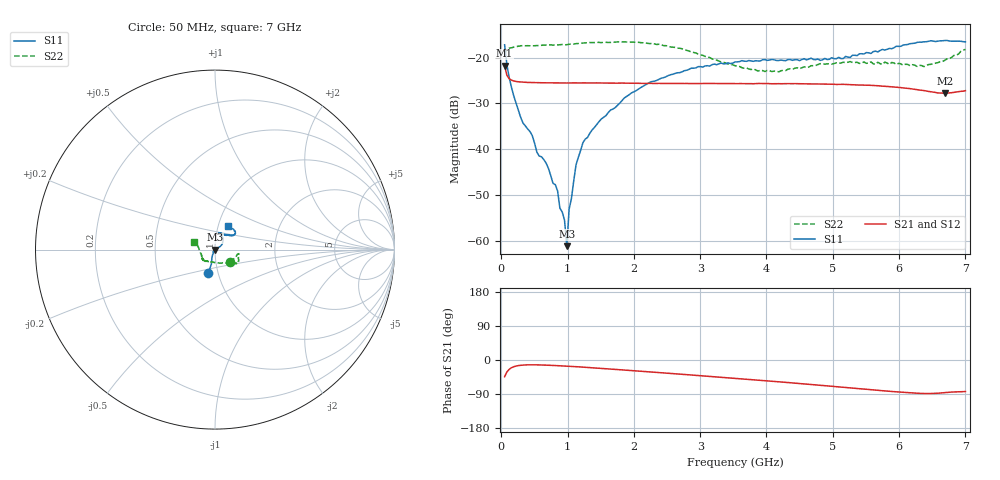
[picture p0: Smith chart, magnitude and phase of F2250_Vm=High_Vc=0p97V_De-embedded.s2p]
! Integrated Device Technology
! Corporate Headquarters
! 6024 Silver Creek Valley Road
! San Jose, CA 95138  USA
! Phone:  1-408-284-8200
! Toll Free:  1-800-223-1366
! Webpage:  http://www.idt.com/
! Timing and RF Division
! 515 Groton Road, Suite 102
! Westford, MA 01886-6024
! Device:  F2250
! Description: Voltage Variable RF Attenuator
! Frequency:  50.0 -  6000.00 MHz
! Package:  3x3 mm Thin QFN Plastic Package: 16 pin
! Ports:  2 RF, 3 DC
!  Pin  1  = GND
!  Pin  2  = NC
!  Pin  3  = RF1  = Port 1
!  Pin  4  = NC
!  Pin  5  = GND
!  Pin  6  = GND
!  Pin  7  = GND
!  Pin  8  = GND
!  Pin  9  = NC
!  Pin 10  = RF2  = Port 2
!  Pin 11  = NC
!  Pin 12  = GND
!  Pin 13  = GND
!  Pin 14  = VCNTRL
!  Pin 15  = VDD
!  Pin 16  = VMODE
! Vcntrl:  0.970 Volts
! Vmode:  +3.300 Volts
! Vdd:  +3.30  Volts
! Current:  1.324 mA
! Data:  The device was measured on a the F2250 evaluation board which has
!  individual transmission lines to the RF pins.  Data was collected
!  using a calibrated network analyzer.  The evaluation board was
!  de-embedded using a TRL calibration technique.
!  The reference plane is the edge of the package pin.
! Misc:  SN 10
!  Action Tracker AT0258
! Date Measured:  2014-11-26
! Date:  2015-10-15  MJV
! Note:
!  Integrated Device Technology supplies this data as a sample of measured
!  data at the package pin for this product.  Your particular data for this
!  product may vary.
!  Data was taken at 25 degrees C.
!  Integrated Device Technology reserves the right to change this data at anytime.
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# GHz S dB R 50
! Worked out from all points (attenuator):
!   201 points, 50 MHz to 7 GHz, reference 50 ohm
!   highest |S21| = -21.78 dB at 50 MHz (marker M1); lowest = -27.8 dB at 6.687 GHz (marker M2)
!   lowest |S11| = -61.1 dB at 988.2 MHz (marker M3), VSWR 1.00, Z = 50.1 - j0.0566 ohm
!   |S11| at or under -10 dB: start of sweep to end of sweep
!   |S22| runs from -23.1 to -16.6 dB; largest |S21 - S12| = 0.00019
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0.05  -17.23 -106.1  -21.78 -44.2  -21.77 -44.2  -19.36 -39.8
0.1195  -24.39 -107.5  -24.62 -24.5  -24.61 -24.5  -17.96 -13.7
0.29325  -33.06 -116.7  -25.32 -14.0  -25.33 -14.0  -17.44 -10.5
0.467  -36.98 -132.7  -25.44 -12.7  -25.46 -12.7  -17.46 -10.9
0.5365  -40.59 -137.1  -25.47 -12.8  -25.47 -12.8  -17.39 -12.3
0.6755  -42.96 -145.0  -25.50 -13.5  -25.48 -13.6  -17.29 -14.3
0.84925  -49.03 178.7  -25.53 -14.9  -25.54 -14.9  -17.25 -17.9
0.884  -52.79 171.2  -25.53 -15.2  -25.55 -15.2  -17.21 -18.8
0.9535  -55.37 -160.4  -25.53 -15.9  -25.53 -15.9  -17.25 -19.6
0.98825  -61.06 -39.6  -25.54 -16.2  -25.53 -16.2  -17.19 -20.1
1.023  -53.04 5.9  -25.53 -16.5  -25.54 -16.5  -17.11 -20.3
1.12725  -43.34 17.8  -25.51 -17.6  -25.54 -17.6  -16.98 -21.9
1.2315  -38.53 19.6  -25.52 -18.8  -25.53 -18.8  -16.82 -23.8
1.857  -28.78 32.3  -25.57 -26.6  -25.57 -26.6  -16.60 -29.8
2.37825  -24.73 42.1  -25.62 -33.2  -25.62 -33.2  -17.10 -34.2
3.525  -20.95 69.7  -25.68 -48.4  -25.68 -48.4  -21.78 -67.4
4.18525  -20.64 76.0  -25.69 -57.5  -25.71 -57.5  -23.12 -106.1
4.7065  -20.43 70.9  -25.73 -65.2  -25.73 -65.2  -21.77 -126.5
5.85325  -18.01 39.4  -26.33 -82.6  -26.34 -82.7  -21.48 -143.4
6.3745  -16.57 40.1  -27.18 -88.4  -27.19 -88.5  -21.98 -163.5
6.68725  -16.29 47.1  -27.79 -86.2  -27.81 -86.3  -20.63 171.8
7  -16.58 61.9  -27.21 -83.3  -27.21 -83.4  -18.22 158.7
